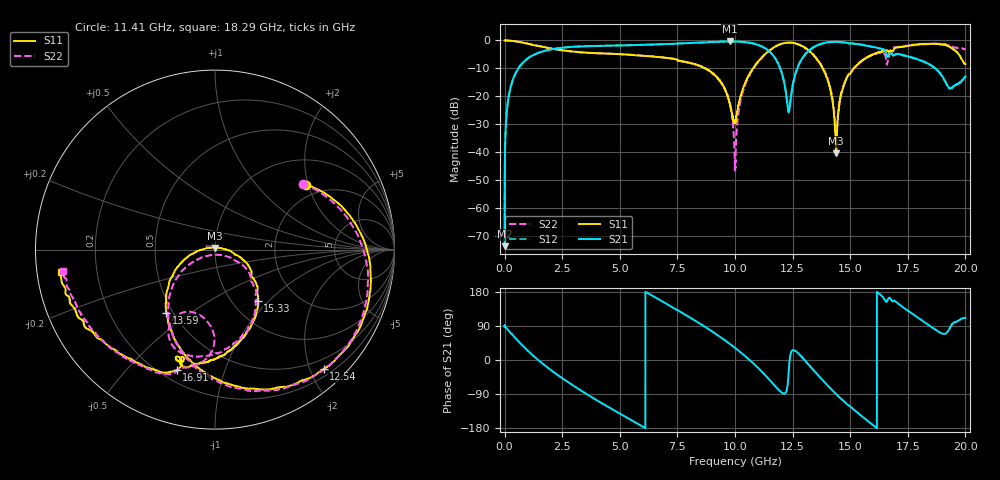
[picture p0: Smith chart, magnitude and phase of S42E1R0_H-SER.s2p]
!{S42E1R0}
!Johanson Technology Inc.
!www.johansontechnology.com
!Test Board Conditions:
!Substrate Type  RO4350B
!Substrate Thickness  50 mil
!Substrate Dk  3.66
!TL Type: GCPW
!TL Trace Width  60 mil
!TL Gap  10 mil
!Electrode orientation  Horizontal
!DUT TOPOLOGY	SERIES
!Mounting Pad LxW  14x55 mil
! Created Wed Nov 25 21:30:34 2020
# khz S ma R 50
! 2 Port Network Data from SP1.SP block
! freq  magS11  angS11  magS21  angS21  magS12  angS12  magS22  angS22
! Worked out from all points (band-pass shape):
!   20001 points, 300 kHz to 20 GHz, reference 50 ohm
!   highest |S21| = -0.36 dB at 9.765 GHz (marker M1); lowest = -73.5 dB at 300 kHz (marker M2)
!   |S21| within 3 dB of the highest: 1.931 GHz to 11.41 GHz (9.48 GHz wide, 142 % of centre); 13.25 GHz to 16.48 GHz (3.232 GHz wide, 21.7 % of centre)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
!   lowest |S11| = -40.3 dB at 14.39 GHz (marker M3), VSWR 1.02, Z = 50 + j0.968 ohm
!   |S11| at or under -10 dB: 8.714 GHz to 10.78 GHz (2.065 GHz wide, 21.2 % of centre); 13.81 GHz to 15.15 GHz (1.346 GHz wide, 9.3 % of centre)
!   |S22| runs from -46.4 to 0.0 dB; largest |S21 - S12| = 0.018
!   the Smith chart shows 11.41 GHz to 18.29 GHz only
!   S11 on the Smith chart (normalised r, x): 11.41 GHz: 1.63, +1.92; 12.54 GHz: 0.32, -2.22; 13.59 GHz: 0.46, -0.40; 15.33 GHz: 1.30, -0.87; 16.91 GHz: 0.26, -0.70; 18.29 GHz: 0.07, -0.07
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300  0.998 -0.2  0.0002108 87.6  0.0002592 80.6  0.9951 -0.0
135300  0.9963 -9.4  0.07661 80.3  0.0772 80.2  0.9966 -9.4
515300  0.9601 -35.2  0.2781 54.8  0.2789 54.9  0.9593 -35.3
1808300  0.7477 -107.0  0.6621 -17.2  0.6638 -17.3  0.744 -107.5
3334300  0.6133 -172.8  0.784 -81.3  0.7827 -81.3  0.6108 -169.8
6667300  0.5055 74.9  0.8536 160.7  0.8515 160.6  0.5094 67.6
8411300  0.3588 9.2  0.9148 98.4  0.9107 98.5  0.3578 8.1
9765300  0.07755 -30.0  0.9598 42.9  0.9597 43.0  0.07719 -47.5
1.00003e7  0.03416 36.7  0.956 32.1  0.959 32.1  0.005156 -124.6
1.04253e7  0.169 82.3  0.9351 11.1  0.9332 11.1  0.1548 102.9
1.14113e7  0.6205 35.6  0.6787 -46.6  0.6745 -46.4  0.6131 36.7
1.23153e7  0.9161 -29.6  0.0536 -44.8  0.05474 -44.2  0.9116 -34.3
1.25413e7  0.8998 -47.7  0.1872 26.0  0.1917 25.5  0.8941 -51.7
1.33343e7  0.5868 -108.9  0.7218 -21.7  0.7211 -22.1  0.594 -108.8
1.35903e7  0.4433 -127.7  0.8252 -39.1  0.8215 -39.2  0.4513 -125.2
1.43893e7  0.009685 87.1  0.9481 -89.9  0.9448 -89.7  0.02925 -89.6
1.53323e7  0.3732 -50.3  0.8598 -139.5  0.8641 -140.0  0.3769 -52.9
1.66673e7  0.6241 -106.8  0.5184 163.3  0.5097 163.0  0.5336 -90.7
1.69053e7  0.7035 -107.6  0.5523 156.7  0.5378 156.6  0.7472 -112.5
1.82893e7  0.8676 -171.8  0.4012 96.9  0.4022 97.9  0.8543 -172.0
1.92903e7  0.7797 136.6  0.1419 80.5  0.1429 79.8  0.8083 142.9
2e7  0.3771 121.0  0.2287 111.6  0.2302 112.5  0.6812 104.0
